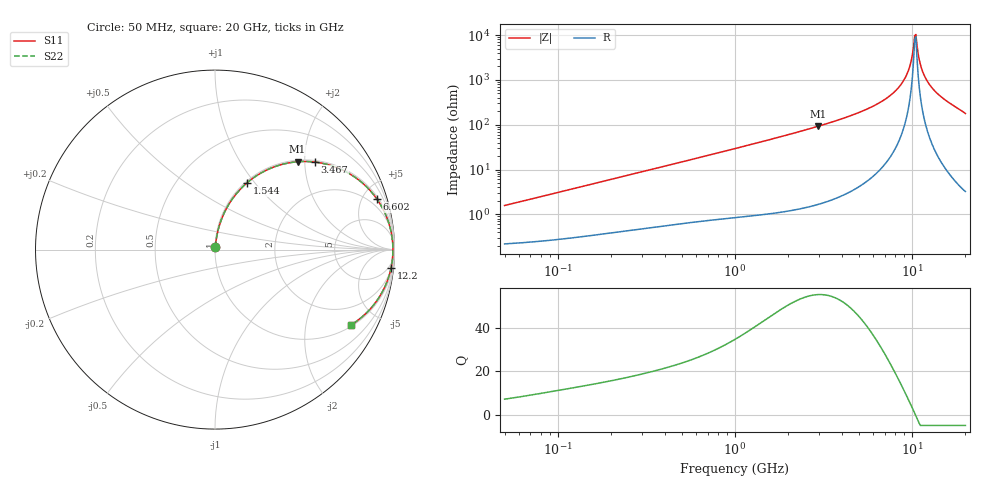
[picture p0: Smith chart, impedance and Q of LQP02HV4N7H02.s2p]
!Murata Part Number: LQP02HV4N7H02
!These Parameters are Measured in Series Mode Connection
!  o--[Z]--o
!Port1  Port2
!  o-------o
!Freq. Start=50[MHz] Stop=20[GHz], 401[Steps]
# Hz S RI R 50
!Freq.(Hz) S11(Real) S11(Imag) S21(Real) S21(Imag) S12(Real) S12(Imag) S22(Real) S22(Imag)
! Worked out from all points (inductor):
!   401 points, 50 MHz to 20 GHz, reference 50 ohm
!   read as one part in series: L = 4.94 nH near 51.52 MHz
!   highest Q = 55.4 at 2.94 GHz (marker M1), where L = 4.99 nH
!   self-resonance near 10.35 GHz
!   S11 on the Smith chart (normalised r, x): 50 MHz: 1.00, +0.03; 1.544 GHz: 1.02, +0.91; 3.467 GHz: 1.04, +2.25; 6.602 GHz: 1.20, +6.30; 12.2 GHz: 2, -19; 20 GHz: 1.06, -3.56
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5e7  0.00243 0.0156  0.9976 -0.0156  0.9976 -0.0156  0.00243 0.0156
1.364002e8  0.00487 0.0412  0.9951 -0.0412  0.9951 -0.0412  0.00487 0.0412
3.721004e8  0.0172 0.108  0.9828 -0.108  0.9828 -0.108  0.0172 0.108
1e9  0.0858 0.2661  0.9142 -0.2661  0.9142 -0.2661  0.0858 0.2661
1.544007e9  0.1783 0.3717  0.8217 -0.3717  0.8217 -0.3717  0.1783 0.3717
2.728004e9  0.4181 0.4842  0.5819 -0.4842  0.5819 -0.4842  0.4181 0.4842
2.940159e9  0.4599 0.4894  0.5401 -0.4894  0.5401 -0.4894  0.4599 0.4894
3.466789e9  0.5568 0.4877  0.4432 -0.4877  0.4432 -0.4877  0.5568 0.4877
4.966507e9  0.7682 0.4112  0.2318 -0.4112  0.2318 -0.4112  0.7682 0.4112
6.601595e9  0.9013 0.2828  0.0987 -0.2828  0.0987 -0.2828  0.9013 0.2828
7.442007e9  0.9414 0.2152  0.0586 -0.2152  0.0586 -0.2152  0.9414 0.2152
8.389408e9  0.9702 0.142  0.0298 -0.142  0.0298 -0.142  0.9702 0.142
9.178299e9  0.9839 0.0845  0.0161 -0.0845  0.0161 -0.0845  0.9839 0.0845
9.745021e9  0.9892 0.0453  0.0108 -0.0453  0.0108 -0.0453  0.9892 0.0453
1.019291e10  0.9912 0.0155  0.00884 -0.0155  0.00884 -0.0155  0.9912 0.0155
1.034674e10  0.9914 0.00559  0.0086 -0.00559  0.0086 -0.00559  0.9914 0.00559
1.066139e10  0.9913 -0.0144  0.00873 0.0144  0.00873 0.0144  0.9913 -0.0144
1.098561e10  0.9903 -0.0344  0.00967 0.0344  0.00967 0.0344  0.9903 -0.0344
1.131968e10  0.9886 -0.0544  0.0114 0.0544  0.0114 0.0544  0.9886 -0.0544
1.220001e10  0.9805 -0.1045  0.0195 0.1045  0.0195 0.1045  0.9805 -0.1045
1.460232e10  0.9389 -0.2227  0.0611 0.2227  0.0611 0.2227  0.9389 -0.2227
2e10  0.7565 -0.4202  0.2435 0.4202  0.2435 0.4202  0.7565 -0.4202
